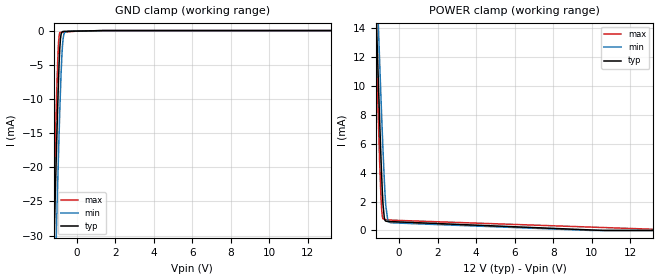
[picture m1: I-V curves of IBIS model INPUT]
|Texas Instruments Incorporated
|THS6301 G.Fast DSL Line Driver
[IBIS Ver]   4.1
[File name]   ths6301.ibs
[Date]   04/05/2018
[File Rev]   1.0
[Source]
| Texas Instruments Incorporated.
| Analog-eLab Design Center, HPA
| 12500 TI Blvd
| Dallas, TX -75243
[Notes]   Revision History:
| Rev 1.0: 04/05/2018
| - Initial version of the model
| - Model generated from simulations in SPECTRE
| - C_comp although listed in numerical order of value are
|   obtained from varying PVT conditions. For PVT conditions for
|   each specific value refer the buffer description under
|   respective [Model]. IBIS model user is responsible for using
|   appropriate C_comp to simulate for Signal Integrity.
[Disclaimer]
| This model is designed as an aid for customers of Texas Instruments.
| TI and its licensors and suppliers make no warranties, either expressed
| or implied, with respect to this  model, including the warranties of
| merchantability or fitness for a particular purpose. The model is
| provided solely on an "as is" basis. The entire risk as to its quality
| and performance is with the customer.
| This model is subject to change without notice. Texas Instruments
| Incorporated is not responsible for updating this model.
[Copyright]
(C) Copyright 2018 Texas Instruments Incorporated.All rights reserved.
|  Component THS6301RSA 16-pin VQFN - RSA package
|  Part # THS6301RSA
[Component]   THS6301RSA
[Manufacturer]  TI
[Package]   |16 VQFN- RSA package
|   typ   min   max
R_pkg   0.1   0.08   0.12
L_pkg   1.0nH   0.8nH   1.2nH
C_pkg   0.2pF   0.16pF   0.24pF
[Pin]   signal_name   model_name   R_pin   L_pin   C_pin
1   IADJ   NC   NA   NA   NA
2   IN+   NC   NA   NA   NA
3   IN-   NC   NA   NA   NA
4   GND   GND   NA   NA   NA
5   NC   NC   NA   NA   NA
6   OUT-   NC   NA   NA   NA
7   B2   INPUT   NA   NA   NA
8   NC   NC   NA   NA   NA
9   NC   NC   NA   NA   NA
10   GND   GND   NA   NA   NA
11   VS   POWER   NA   NA   NA
12   NC   NC   NA   NA   NA
13   NC   NC   NA   NA   NA
14   NC   NC   NA   NA   NA
15   OUT+   NC   NA   NA   NA
16   B1   INPUT   NA   NA   NA
| Models and submodels in the file (1): INPUT (Input)
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|   Model INPUT
[Model]   INPUT
Model_type   Input
Vinl = 0.6
Vinh = 2.3
|   typ   min   max
|   (nom PVT)   (fast PVT)   (slow PVT)
C_comp   0.307p   0.300p   0.308p
[Voltage Range]   12   11.4   12.6
[Temperature Range]   27   125   -40
[Power Clamp Reference]   12   11.4   12.6
[GND Clamp Reference]   0   0   0
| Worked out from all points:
|   GND clamp passes 1 mA (typ) near -0.83 V on its own axis
|   POWER clamp passes 1 mA (typ) near -0.78 V on its own axis
[GND Clamp]
|   Voltage   I(typ)   I(min)   I(max)
-12V      -1.372A    -1.381A    -1.367A
-1.236V   -38.38mA   -50.34mA   -30.76mA
-1.164V   -30.21mA   -42.15mA   -22.59mA
-1.056V   -18.35mA   -30.11mA   -11.02mA
-984mV    -11.22mA   -22.5mA    -4.471mA
-948mV    -7.803mA   -18.76mA   -2.102mA
-876mV    -2.641mA   -11.85mA   -289.1uA
-840mV    -1.183mA   -8.741mA   -280.4uA
-732mV    -152.6uA   -2.064mA   -254.4uA
-660mV    -117.9uA   -511uA     -237.2uA
-444mV    -103uA     -96.48uA   -185.3uA
24V       0A         0A         0A
[POWER Clamp]
|   Voltage   I(typ)   I(min)   I(max)
-12V      587.8mA    539.9mA    628.2mA
-1.236V   16.94mA    20.27mA    14.55mA
-1.128V   12.32mA    16.05mA    9.807mA
-1.056V   9.355mA    13.32mA    6.643mA
-948mV    5.174mA    9.33mA     2.46mA
-912mV    3.915mA    8.05mA     1.528mA
-840mV    1.852mA    5.609mA    805uA
-768mV    844.7uA    3.43mA     777.4uA
-696mV    646.6uA    1.754mA    749.8uA
-588mV    622.9uA    678.5uA    731.5uA
-444mV    614.6uA    536.4uA    722.6uA
24V       0A         0A         0A
